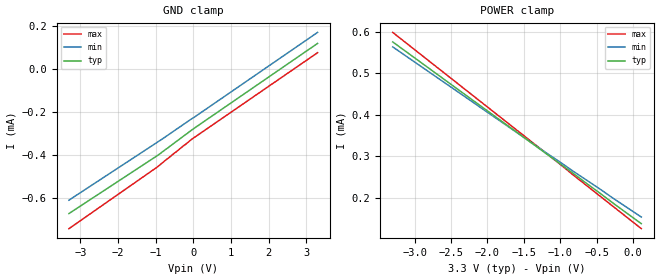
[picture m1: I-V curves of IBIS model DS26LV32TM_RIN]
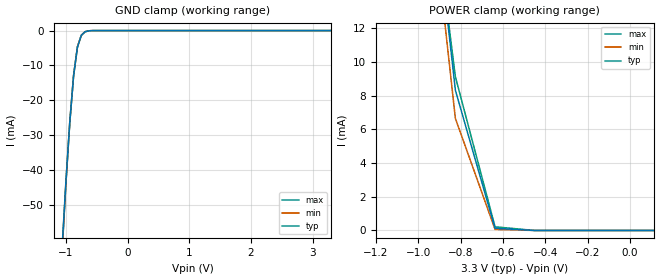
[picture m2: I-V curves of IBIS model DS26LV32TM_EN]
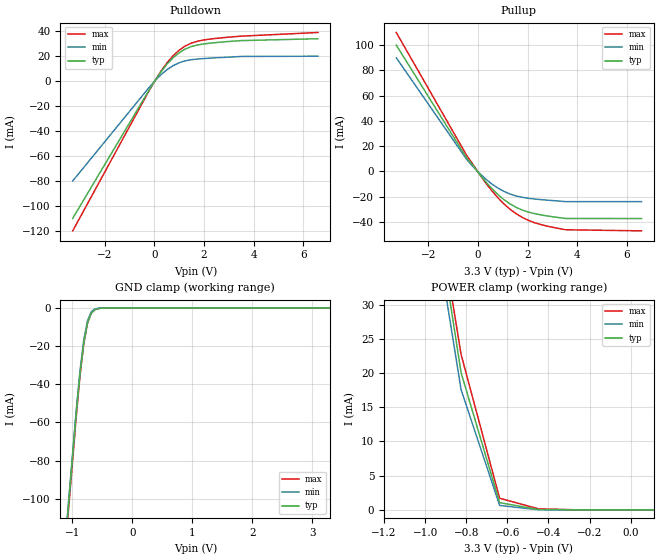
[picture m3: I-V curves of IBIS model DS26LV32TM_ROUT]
|   National Semiconductor Corporation
|   Interface Products Group
|   IBIS Model of DS26LV32TM
|   16L SOIC Package
[IBIS Ver]   2.1
[File name]   26lv32tm.ibs
[File Rev]   1.2
[Date]   12/17/2001
[Source]   File originated at National Semiconductor Corporation.
   Interface Group/Analog Division group. All data based on
   Empirical Measurements(Bench).
[Notes]   File created by MS, TL & SBH.
   Rev 1.2, removed C_comp min and max values
   C_comp should only have typical value---milt
[Disclaimer]
(C) Copyright National Semiconductor Corporation 1994
   All rights reserved
   National Semiconductor Corporation hereby grants
the user of this IBIS model a non-exclusive, nontransferable
license to use this IBIS model under the following terms.
Before using this IBIS model, the user should read this
license.  If the user does not accept these terms,  the
IBIS model should be returned to National within 30 days.
   The user is granted this license only to use the
IBIS model and is not granted rights to sell, load, rent,
lease or license the IBIS model in whole or in part, or in
modified form to anyone other than user. User may modify
the IBIS model to suit its specific applications but rights
to derivative works and such modifications shall belong to
National.
   This IBIS model is provided on an "AS IS" basis and
National makes absolutely no warranty with respect to the
information contained herein.NATIONAL DISCLAIMS AND CUSTOMER
WAIVES ALL WARRANTIES, EXPRESS OR IMPLIED, INCLUDING
WARRANTIES OF MERCHANTABILITY OR FITNESS FOR A PARTICULAR
PURPOSE. The entire risk as to quality and performance is
with the Customer. ACCORDINGLY, IN NO EVENT SHALL THE
COMPANY BE LIABLE FOR ANY DAMAGES, WHETHER IN CONTRACT OR
TORT,INCLUDING ANY LOST PROFITS OR OTHER INCIDENTAL,
CONSEQUENTIAL, EXEMPLARY, OR PUNITIVE DAMAGES ARISING OUT
OF THE USE OR APPLICATION OF THE IBIS model provided in
this package.Further, National reserves the right to make
changes without notice to any product herein to improve
reliability, function, or design. National does not convey
any license under patent rights or any other intellectual
property rights, including those of third parties.
   National is not obligated to provide maintenance or support
for the licensed IBIS model.
Contact National at ATTN:INTERFACE APPLICATIONS/IBIS MODELS.
2900 Semiconductor Drive, M/S A2595, Santa Clara, CA 95052-8090
[Copyright]   Copyright 1994, National Semiconductor, All Rights Reserved
[Component]   DS26LV32TM
[Manufacturer]  National Semiconductor Corp
[Package]
|   typ   min   max
R_pkg   50.0m   NA   NA
L_pkg   1.37nH   NA   NA
C_pkg   0.26pF   NA   NA
[Pin]   signal_name   model_name   R_pin   L_pin   C_pin
1   RINA-   DS26LV32TM_RIN   50.0m   2.07n   0.429p
2   RINA+   DS26LV32TM_RIN   50.0m   1.49n   0.306p
3   ROUTA   DS26LV32TM_ROUT   50.0m   0.95n   0.146p
4   EN   DS26LV32TM_EN   50.0m   0.95n   0.152p
5   ROUTC   DS26LV32TM_ROUT   50.0m   0.95n   0.152p
6   RINC+   DS26LV32TM_RIN   50.0m   0.95n   0.146p
7   RINC-   DS26LV32TM_RIN   50.0m   1.49n   0.306p
8   GND   GND   50.0m   2.07n   0.429p
9   RIND-   DS26LV32TM_RIN   50.0m   2.07n   0.429p
10   RIND+   DS26LV32TM_RIN   50.0m   1.49n   0.306p
11   ROUTD   DS26LV32TM_ROUT   50.0m   0.95n   0.146p
12   EN*   DS26LV32TM_EN   50.0m   0.95n   0.152p
13   ROUTB   DS26LV32TM_ROUT   50.0m   0.95n   0.152p
14   RINB+   DS26LV32TM_RIN   50.0m   0.95n   0.146p
15   RINB-   DS26LV32TM_RIN   50.0m   1.49n   0.306p
16   VCC   POWER   50.0m   2.07n   0.429p
[Diff_pin]   inv_pin   vdiff   tdelay_typ   tdelay_min   tdelay_max
| The '+' pin is Diff_pin and the '-' pin is the inv_pin
2   1   0.1   0 0 0  | Receiver Vth=+/-100mV
6   7   0.1   0 0 0
10   9   0.1   0 0 0
14   15   0.1   0 0 0
| Models and submodels in the file (3): DS26LV32TM_RIN (Input), DS26LV32TM_EN (Input), DS26LV32TM_ROUT (3-state)
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|   Receiver Input  MODEL
[Model]   DS26LV32TM_RIN
Model_type   Input
|Signals   RINA-,RINA+,RINC+,RINC-,RIND-,RIND+,RINB+,RINB-
Vinh = 2.0
Vinl = 0.8
|   typ   min   max
C_comp   4.508pF   NA   NA
|   typ   min   max
[Temperature Range]   25.0   NA   NA
[Voltage range]   3.3V   3.0V   3.6V
[Power_clamp]
| Note that the[POWER_clamp]voltage table is referenced to Vcc
| and is calculated using Vtable=Vcc - Vmeasured.
| Receiver Inputs do not have Power Clamp
|  Voltage   I(typ)   I(min)   I(max)
-3.3V     576uA      564uA      599uA
-1.2V     307uA      309uA      308uA
-1.012V   283uA      287uA      282uA
-825mV    259uA      264uA      255uA
-637.5mV  234uA      242uA      229uA
-450mV    210uA      220uA      203uA
-262.5mV  185uA      197uA      177uA
-75mV     161uA      175uA      151uA
112.5mV   137uA      153uA      125uA
[GND_clamp]
|  Voltage   I(typ)   I(min)   I(max)
-3.3V     -670uA     -608uA     -740uA
-958.3mV  -402uA     -340uA     -455uA
-41.67mV  -283uA     -231uA     -326uA
3.3V      118uA      169uA      75uA
|   Receiver Enable  MODEL
[Model]   DS26LV32TM_EN
Model_type   Input
|Signals   EN,EN*
Vinh = 2.0
Vinl = 0.8
|   typ   min   max
C_comp   1.877pF   NA   NA
|   typ   min   max
[Temperature Range]   25.0   NA   NA
[Voltage range]   3.3V   3.0V   3.6V
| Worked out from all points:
|   GND clamp passes 1 mA (typ) near -0.73 V on its own axis
|   POWER clamp passes 1 mA (typ) near -0.66 V on its own axis
[GND_clamp]
|  Voltage   I(typ)   I(min)   I(max)
-3.3V     -630mA     -630mA     -630mA
-1.062V   -62.66mA   -63.7mA    -64.17mA
-1V       -43.49mA   -43.95mA   -44.13mA
-937.5mV  -26.45mA   -26.46mA   -26.71mA
-875mV    -12.97mA   -12.81mA   -13.02mA
-812.5mV  -4.741mA   -4.629mA   -4.699mA
-750mV    -1.383mA   -1.354mA   -1.337mA
-687.5mV  -337uA     -338uA     -315uA
-500mV    -712nA     -773nA     -712nA
3.3V      0A         0A         0A
[Power_clamp]
| Note that the[POWER_clamp]voltage table is referenced to Vcc
| and is calculated using Vtable=Vcc - Vmeasured.
| No Power Clamp for Enable inputs
|  Voltage   I(typ)   I(min)   I(max)
-3.3V     456mA      456mA      456mA
-1.2V     58.63mA    51.17mA    55.03mA
-1.012V   29.48mA    28.02mA    27.88mA
-825mV    8.33mA     6.658mA    9.135mA
-637.5mV  129uA      62.7uA     216uA
-450mV    107nA      47.1nA     217nA
-262.5mV  140pA      302pA      208pA
-75mV     169pA      102pA      -92pA
112.5mV   192pA      -78.3pA    -200pA
|   Receiver Output  MODEL
[Model]   DS26LV32TM_ROUT
Model_type   3-state
| Signals   ROUTA,ROUTB,ROUTC,ROUTD
Vmeas = 1.5V   |Reference voltage is at 50% of output swing
Cref = 15pF   |Timing specification test load capacitance value
Vref = 0   |Timing specification test load voltage; GND
| variable   typ   min   max
C_comp   3.09pF   NA   NA
|   typ   min   max
[Temperature Range]   25.0   NA   NA
[Voltage range]   3.3V   3.0V   3.6V
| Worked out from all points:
|   slope of the pulldown table from 0 to 0.495 V, typ, clamps not added: 36.5 ohm
|   slope of the pullup table from 0 to 0.495 V, typ, clamps not added: 42.5 ohm
|   GND clamp passes 1 mA (typ) near -0.62 V on its own axis
|   POWER clamp passes 1 mA (typ) near -0.63 V on its own axis
[Pulldown]
|  Voltage   I(typ)   I(min)   I(max)
-3.3V     -110mA     -80mA      -120mA
0V        -224uA     -118uA     -267uA
500mV     13.46mA    9.097mA    14.54mA
750mV     18.73mA    12.39mA    20.33mA
1V        22.83mA    14.77mA    24.88mA
1.25V     25.81mA    16.31mA    28.25mA
1.5V      27.82mA    17.22mA    30.56mA
2.25V     30.47mA    18.47mA    33.73mA
3.5V      32.51mA    19.79mA    36.06mA
6.6V      34mA       20mA       39mA
[Pullup]
| Note that the[Pullup]voltage table is referenced to Vcc
| and is calculated using Vtable=Vcc - Vmeasured.
|   Voltage   I(typ)   I(min)   I(max)
-3.3V     100mA      90mA       110mA
-450mV    10.47mA    9.334mA    12.45mA
-200mV    4.833mA    3.805mA    5.52mA
50mV      -1.858mA   -1.3mA     -1.914mA
550mV     -13.38mA   -9.767mA   -15.08mA
800mV     -18.22mA   -13.1mA    -20.75mA
1.3V      -25.75mA   -17.89mA   -29.99mA
1.8V      -30.63mA   -20.5mA    -36.49mA
2.3V      -33.44mA   -21.82mA   -40.66mA
3.55V     -37.2mA    -23.89mA   -46.13mA
6.6V      -37.27mA   -23.89mA   -47mA
[GND_clamp]
| Outputs in Tri-state.
|  Voltage   I(typ)   I(min)   I(max)
-3.3V     -935mA     -935mA     -935mA
-1V       -78.2mA    -77.62mA   -81.35mA
-937.5mV  -55.13mA   -53.96mA   -57.3mA
-875mV    -34.77mA   -33.3mA    -36.07mA
-812.5mV  -18.66mA   -17.15mA   -19.25mA
-750mV    -8.034mA   -6.89mA    -8.198mA
-687.5mV  -2.862mA   -2.151mA   -2.82mA
-625mV    -1.011mA   -600uA     -926uA
-562.5mV  -405uA     -174uA     -336uA
-375mV    -5.49uA    -644nA     -3.32uA
3.3V      0A         0A         0A
[POWER_clamp]
| Note that the[POWER_clamp]voltage table is referenced to Vcc
| and is calculated using Vtable=Vcc - Vmeasured.
| Outputs in Tri-state.
|Voltage   I(typ)   I(min)   I(max)
-3.3V     595mA      595mA      595mA
-1.2V     88.89mA    80.96mA    90.46mA
-1.012V   56.51mA    52.66mA    57.48mA
-825mV    20.05mA    17.57mA    22.71mA
-637.5mV  1.051mA    645uA      1.694mA
-450mV    54.9uA     15.9uA     158uA
-262.5mV  157nA      22.1nA     1.46uA
-75mV     231pA      124pA      1.65nA
112.5mV   200pA      221pA      -212pA
[Ramp]
|   typ   min   max
dV/dt_r   1.89/1.68n   1.74/2.44n   2.09/1.38n
dV/dt_f   1.9/1.73n   1.72/2.43n   2.1/1.43n
R_load = 1MOhm   | Represents an open
